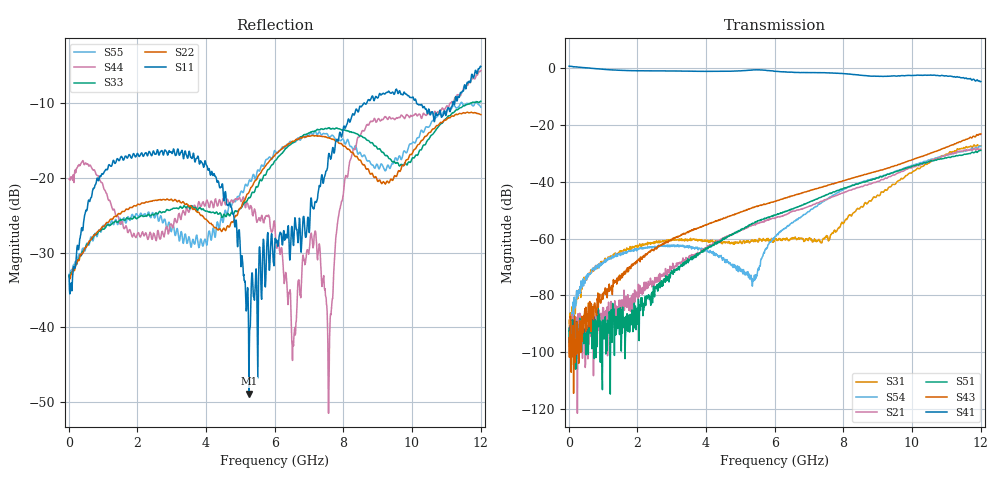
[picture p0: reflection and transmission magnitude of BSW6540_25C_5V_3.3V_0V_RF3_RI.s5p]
! Agilent Technologies	N5230C	MY49001333	A.09.33.09
!	Test time	=	2026-05-06 10:00
!	Product	=	BSW6540
!	Temp	=	25C
!	VDD	=	5
!	Control_High	=	3.3
!	Control_Low	=	0
!	Logic	=	RF3
!	Port1	=	RFC
!	Port2	=	RF1
!	Port3	=	RF2
!	Port4	=	RF3
!	Port5	=	RF4
!	V1	=	3.3 / 0
!	V2	=	3.3 / 0
!S5P File: Measurements: <S11,S12,S13,S14,S15>,
!<S21,S22,S23,S24,S25>,
!<S31,S32,S33,S34,S35>,
!<S41,S42,S43,S44,S45>,
!<S51,S52,S53,S54,S55>;
# HZ S RI R 50
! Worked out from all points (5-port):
!   1201 points, 10 MHz to 12.01 GHz, reference 50 ohm
!   strongest paths, dB at 10 MHz, 3.01 GHz, 6.01 GHz, 9.01 GHz, 12.01 GHz:
!     S41: 0.6, -1.1, -1.2, -3.0, -4.8
!     S43: -94.9, -60.5, -46.9, -36.2, -23.2
!     S51: -96.4, -72.2, -51.8, -38.7, -29.0
!     S21: -100.4, -70.0, -53.0, -39.9, -28.6
!     S54: -92.6, -62.5, -59.2, -38.6, -27.5
!     S31: -97.8, -60.5, -60.2, -44.7, -27.5
!   lowest |S11| = -48.9 dB at 5.25 GHz (marker M1), VSWR 1.01, Z = 50.2 + j0.267 ohm
!   |S11| at or under -10 dB: start of sweep to 8.602 GHz; 8.619 GHz to 8.683 GHz (63.64 MHz wide, 0.736 % of centre); 10.14 GHz to 11.19 GHz (1.051 GHz wide, 9.86 % of centre)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
